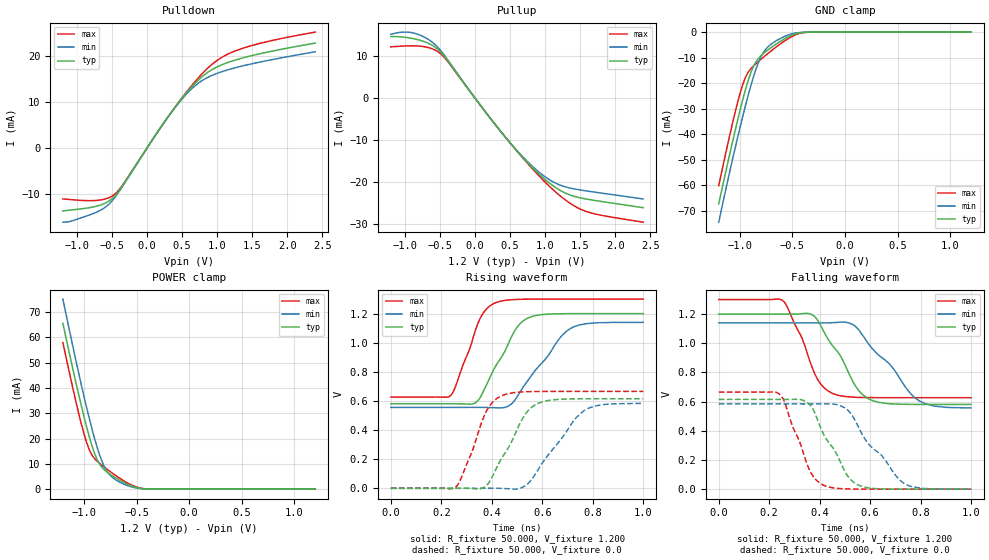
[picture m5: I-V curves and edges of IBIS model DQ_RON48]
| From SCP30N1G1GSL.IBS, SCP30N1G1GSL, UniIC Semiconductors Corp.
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|   Model DQ_RON48
[Model] DQ_RON48
Model_type I/O
Vinl =  0.500V
Vinh =  0.700V
Vmeas =  0.600V
Rref =  50.000
Vref =  0.600V
C_comp   1.373pF   1.353pF   1.403pF
[Model Spec]
Vinh   0.700V   0.670V   0.750V
Vinl   0.500V   0.470V   0.550V
Vmeas   0.600V   0.570V   0.650V
Vref   0.600V   0.570V   0.650V
Rref   50.000   NA   NA
[Temperature Range]   25.000   85.000   -40.000
[Voltage Range]   1.200V   1.140V   1.300V
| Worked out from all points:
|   slope of the pulldown table from 0 to 0.18 V, typ, clamps not added: 43.2 ohm
|   slope of the pullup table from 0 to 0.18 V, typ, clamps not added: 45.2 ohm
|   GND clamp passes 1 mA (typ) near -0.49 V on its own axis
|   POWER clamp passes 1 mA (typ) near -0.53 V on its own axis
|   rising waveform, R_fixture 50.000, V_fixture 1.200: 20-80 % time 112ps typ, 150ps min, 84.6ps max; typ from 0.581 V to 1.2 V
|   rising waveform, R_fixture 50.000, V_fixture 0.0: 20-80 % time 112ps typ, 146ps min, 86.4ps max; typ from 0 V to 0.615 V
|   falling waveform, R_fixture 50.000, V_fixture 1.200: 20-80 % time 125ps typ, 169ps min, 96.5ps max; typ from 1.2 V to 0.581 V
|   falling waveform, R_fixture 50.000, V_fixture 0.0: 20-80 % time 111ps typ, 150ps min, 86.1ps max; typ from 0.615 V to 0 V
[Pulldown]
|Voltage   I(typ)   I(min)   I(max)
-1.2V     -13.75mA   -16.21mA   -11.13mA
-719mV    -12.71mA   -14.02mA   -11.45mA
-571mV    -11.85mA   -12.65mA   -11.03mA
-460mV    -10.51mA   -10.84mA   -10.1mA
-349mV    -8.251mA   -8.358mA   -8.093mA
317mV     7.181mA    7.145mA    7.169mA
576mV     12.31mA    12.01mA    12.49mA
761mV     15.26mA    14.49mA    15.82mA
1.02V     17.87mA    16.43mA    19.36mA
1.279V    19.31mA    17.62mA    21.34mA
1.723V    20.98mA    19.13mA    23.28mA
2.4V      22.93mA    21.03mA    25.33mA
[Pullup]
|Voltage   I(typ)   I(min)   I(max)
-1.2V     14.6mA     15.17mA    12.16mA
-1.004V   14.45mA    15.68mA    12.37mA
-819mV    13.89mA    15.18mA    12.37mA
-634mV    12.76mA    13.59mA    11.85mA
-486mV    10.89mA    11.24mA    10.48mA
69mV      -1.544mA   -1.554mA   -1.522mA
439mV     -9.432mA   -9.411mA   -9.404mA
772mV     -15.74mA   -15.49mA   -15.95mA
1.031V    -19.81mA   -19.1mA    -20.49mA
1.29V     -22.61mA   -21.13mA   -24.26mA
1.549V    -23.9mA    -21.99mA   -26.74mA
2.4V      -26.08mA   -24.02mA   -29.54mA
[GND_clamp]
|Voltage   I(typ)   I(min)   I(max)
-1.2V     -67.26mA   -74.42mA   -60.1mA
-1.05V    -39.62mA   -46.47mA   -32.4mA
-1V       -31.05mA   -37.77mA   -24.37mA
-950mV    -23.16mA   -29.46mA   -18.1mA
-925mV    -19.62mA   -25.5mA    -16.02mA
-875mV    -13.89mA   -18.21mA   -13.48mA
-825mV    -10.4mA    -12.16mA   -11.61mA
-775mV    -8.365mA   -7.964mA   -9.852mA
-700mV    -6.001mA   -4.671mA   -7.319mA
-525mV    -1.587mA   -933.3uA   -2.208mA
-375mV    -90.13uA   -49.22uA   -132.9uA
1.2V      0A         0A         0A
[POWER_clamp]
|Voltage   I(typ)   I(min)   I(max)
-1.2V     65.51mA    75.11mA    57.91mA
-1.05V    37.38mA    45.87mA    29.99mA
-1V       28.74mA    36.73mA    21.95mA
-950mV    20.85mA    28.08mA    15.65mA
-925mV    17.34mA    24.01mA    13.56mA
-875mV    11.74mA    16.61mA    11.06mA
-825mV    8.457mA    10.65mA    9.317mA
-775mV    6.603mA    6.7mA      7.708mA
-725mV    5.177mA    4.492mA    6.178mA
-550mV    1.336mA    943.1uA    1.707mA
-400mV    85.95uA    67.55uA    91.19uA
1.2V      0A         0A         0A
[Ramp]
| variable   typ   min   max
dV/dt_r   0.369/0.112n   0.350/0.146n   0.400/86.560p
dV/dt_f   0.372/0.125n   0.350/0.169n   0.404/96.543p
R_load = 50.000
[Rising Waveform]
R_fixture= 50.000
V_fixture= 1.200
V_fixture_min= 1.140
V_fixture_max= 1.300
|time   V(typ)   V(min)   V(max)
0s        580.6mV    556mV      627mV
233ps     580.7mV    556mV      631.4mV
255ps     580.6mV    556mV      693.3mV
339ps     592.4mV    556.1mV    1.105V
376ps     700.4mV    555.5mV    1.226V
418ps     847.3mV    553.2mV    1.276V
478ps     1.04V      580.1mV    1.295V
531ps     1.158V     712.2mV    1.299V
714ps     1.2V       1.1V       1.3V
1ns       1.2V       1.14V      1.3V
[Rising Waveform]
R_fixture= 50.000
V_fixture= 0.0
V_fixture_min= 0.0
V_fixture_max= 0.0
|time   V(typ)   V(min)   V(max)
0s        42.45nV    135.7nV    24.88nV
259ps     100.6uV    -6.978uV   11.35mV
321ps     -1.418mV   -13.13uV   248.2mV
372ps     9.306mV    164.6uV    506.1mV
406ps     93.07mV    431.6uV    595.9mV
443ps     217.7mV    -774uV     638.2mV
530ps     502.5mV    14.11mV    662.8mV
588ps     586.8mV    140.2mV    665.2mV
764ps     615mV      532mV      665.9mV
1ns       615.4mV    583.8mV    665.9mV
[Falling Waveform]
R_fixture= 50.000
V_fixture= 1.200
V_fixture_min= 1.140
V_fixture_max= 1.300
|time   V(typ)   V(min)   V(max)
0s        1.2V       1.14V      1.3V
256ps     1.2V       1.14V      1.29V
331ps     1.203V     1.14V      1.031V
375ps     1.19V      1.14V      812.6mV
414ps     1.088V     1.14V      701.2mV
452ps     980.9mV    1.141V     656mV
530ps     742.8mV    1.13V      631.1mV
606ps     609.9mV    968.1mV    627.6mV
793ps     580.9mV    606.9mV    627mV
1ns       580.6mV    556.5mV    627mV
[Falling Waveform]
R_fixture= 50.000
V_fixture= 0.0
V_fixture_min= 0.0
V_fixture_max= 0.0
|time   V(typ)   V(min)   V(max)
0s        615.4mV    584mV      665.9mV
244ps     615.3mV    584.1mV    646.6mV
259ps     615.3mV    584.1mV    605.6mV
357ps     585.6mV    583.9mV    141.8mV
388ps     491.2mV    584mV      59.33mV
424ps     349.3mV    584.8mV    20.99mV
508ps     97.67mV    546.7mV    1.832mV
564ps     20.55mV    390.4mV    361.4uV
732ps     166.1uV    41.81mV    2.709uV
1ns       105.3nV    26.11uV    17.29nV
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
